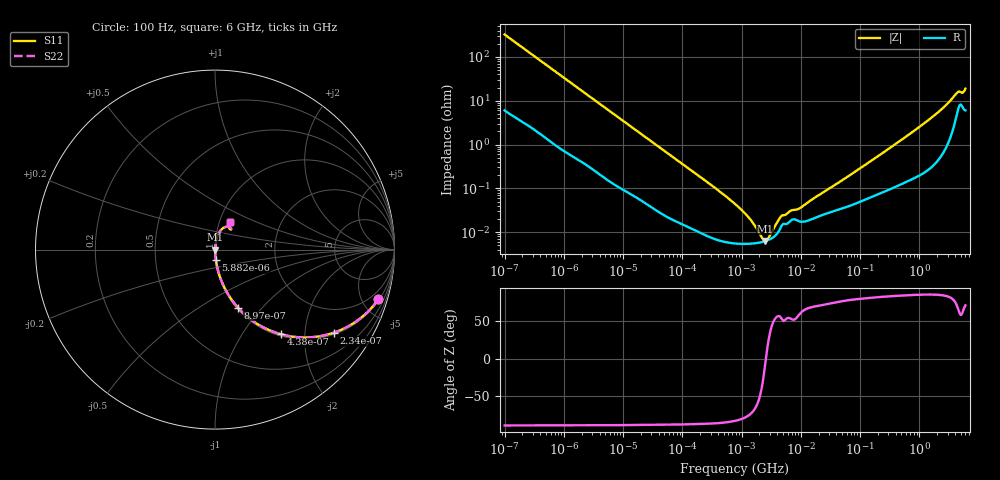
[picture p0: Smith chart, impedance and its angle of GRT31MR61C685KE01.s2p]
!Murata Part Number: GRT31MR61C685KE01
!These Parameters are Measured in Series Mode Connection
!Data Generated on Jun 19, 2026
!  o--ll--o
!Port1  Port2
!  o------o
!Operation Temp=25[degC], DC Bias Voltage=0[V]
!Freq. Start=100[Hz] Stop=6[GHz] 401[Steps]
# Hz S RI R 50
!Freq.(Hz) S11(Real) S11(Imag) S21(Real) S21(Imag) S12(Real) S12(Imag) S22(Real) S22(Imag)
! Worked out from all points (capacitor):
!   401 points, 100 Hz to 6 GHz, reference 50 ohm
!   read as one part in series: C = 4.86 uF near 109 Hz
!   lowest |Z| = 6.31 mohm at 2.481 MHz (marker M1)
!   series resonance near 2.573 MHz, so ESL is about 790 pH
!   S11 on the Smith chart (normalised r, x): 100 Hz: 1.12, -6.52; 234 Hz: 1.06, -2.81; 438 Hz: 1.03, -1.52; 897 Hz: 1.02, -0.75; 5.882 kHz: 1.00, -0.12; 6 GHz: 1.12, +0.36
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100  0.9098 -0.2774  0.0902 0.2774  0.0902 0.2774  0.9098 -0.2774
150  0.8227 -0.3724  0.1773 0.3724  0.1773 0.3724  0.8227 -0.3724
234  0.6614 -0.4632  0.3386 0.4632  0.3386 0.4632  0.6614 -0.4632
438  0.368 -0.4719  0.632 0.4719  0.632 0.4719  0.368 -0.4719
897  0.1278 -0.3235  0.8722 0.3235  0.8722 0.3235  0.1278 -0.3235
2008  0.0314 -0.1629  0.9686 0.1629  0.9686 0.1629  0.0314 -0.1629
5882  0.00485 -0.0582  0.9951 0.0582  0.9951 0.0582  0.00485 -0.0582
40335  0.000364 -0.00883  0.9996 0.00883  0.9996 0.00883  0.000364 -0.00883
774597  5.54e-05 -0.000439  0.9999 0.000439  0.9999 0.000439  5.54e-05 -0.000439
1267578  5.43e-05 -0.000224  0.9999 0.000224  0.9999 0.000224  5.43e-05 -0.000224
1896632  5.72e-05 -9.09e-05  0.9999 9.09e-05  0.9999 9.09e-05  5.72e-05 -9.09e-05
2481164  6.22e-05 -1.07e-05  0.9999 1.07e-05  0.9999 1.07e-05  6.22e-05 -1.07e-05
3245845  7.3e-05 7.07e-05  0.9999 -7.07e-05  0.9999 -7.07e-05  7.3e-05 7.07e-05
4246196  0.000105 0.000162  0.9999 -0.000162  0.9999 -0.000162  0.000105 0.000162
4856642  0.000148 0.000191  0.9999 -0.000191  0.9999 -0.000191  0.000148 0.000191
6948629  0.000189 0.000251  0.9998 -0.000251  0.9998 -0.000251  0.000189 0.000251
9506416  0.000177 0.000301  0.9998 -0.000301  0.9998 -0.000301  0.000177 0.000301
1.555665e7  0.0002 0.000525  0.9998 -0.000525  0.9998 -0.000525  0.0002 0.000525
3.124326e8  0.00101 0.00815  0.999 -0.00815  0.999 -0.00815  0.00101 0.00815
1.712697e9  0.00519 0.0436  0.9948 -0.0436  0.9948 -0.0436  0.00519 0.0436
4.193612e9  0.0571 0.1259  0.9429 -0.1259  0.9429 -0.1259  0.0571 0.1259
6e9  0.0833 0.1552  0.9167 -0.1552  0.9167 -0.1552  0.0833 0.1552
